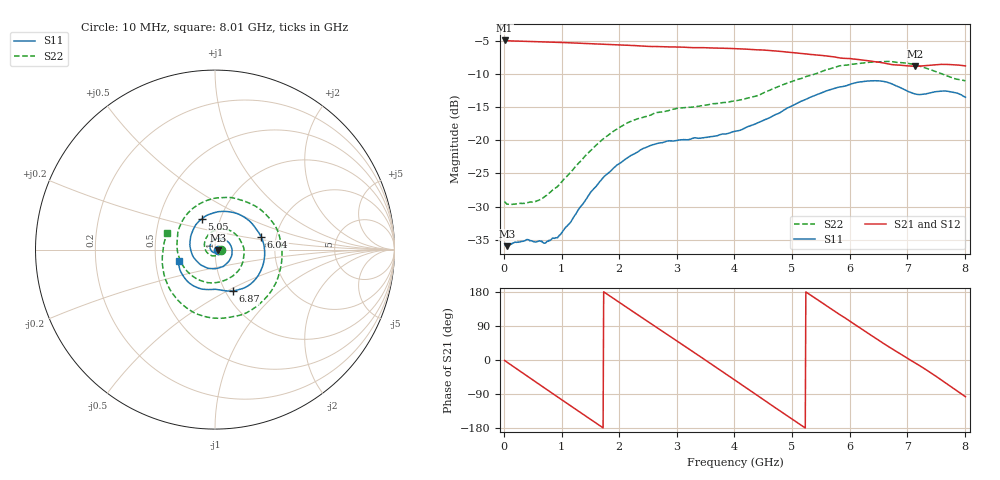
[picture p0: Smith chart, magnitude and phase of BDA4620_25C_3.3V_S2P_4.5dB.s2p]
!Agilent Technologies,E5071B,MY42404982,A.09.10
!Date: Wed May 06 08:56:56 2026
!Data & Calibration Information:
!Freq	S11:SOLT2(ON)	S21:SOLT2(ON)	S12:SOLT2(ON)	S22:SOLT2(ON)
# Hz S RI R 50
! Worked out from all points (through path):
!   801 points, 10 MHz to 8.01 GHz, reference 50 ohm
!   highest |S21| = -4.95 dB at 10 MHz (marker M1); lowest = -8.8 dB at 7.14 GHz (marker M2)
!   group delay of S21, straight-line fit = 283 ps
!   lowest |S11| = -36.0 dB at 60 MHz (marker M3), VSWR 1.03, Z = 51.6 - j0.143 ohm
!   |S11| at or under -10 dB: start of sweep to end of sweep
!   |S22| runs from -29.7 to -8.1 dB; largest |S21 - S12| = 0.0027
!   S11 on the Smith chart (normalised r, x): 10 MHz: 1.03, -0.00; 5.05 GHz: 0.82, +0.29; 6.04 GHz: 1.67, +0.26; 6.87 GHz: 1.08, -0.53; 8.01 GHz: 0.66, -0.08
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1e7  0.0166 -0.000983  0.5656 -0.0118  0.5661 -0.0123  0.0344 -0.00275
6e7  0.0158 -0.00139  0.5596 -0.0645  0.5608 -0.0654  0.0325 -0.0058
3.7e8  0.0143 -0.0101  0.4328 -0.3513  0.4332 -0.3522  0.0191 -0.0275
7.3e8  -8.32e-05 -0.017  0.1274 -0.5364  0.127 -0.5372  -0.0173 -0.0341
1.03e9  -0.0188 -0.00905  -0.1668 -0.5192  -0.1675 -0.5198  -0.0495 -0.0093
1.35e9  -0.0279 0.0165  -0.4186 -0.3392  -0.4189 -0.3394  -0.0573 0.0423
1.64e9  -0.0156 0.0447  -0.5251 -0.0844  -0.5256 -0.085  -0.0282 0.0909
1.93e9  0.0155 0.0614  -0.4913 0.1847  -0.4917 0.1851  0.0326 0.1147
2.32e9  0.0663 0.0476  -0.253 0.4497  -0.2537 0.4499  0.1226 0.078
2.68e9  0.0951 -0.000848  0.0618 0.5045  0.0626 0.505  0.162 -0.00966
3.38e9  0.0345 -0.0975  0.4891 0.102  0.4897 0.101  0.0451 -0.1747
3.69e9  -0.0225 -0.1055  0.4651 -0.1705  0.4647 -0.1718  -0.0666 -0.1771
4.01e9  -0.0835 -0.0815  0.2931 -0.3931  0.293 -0.3939  -0.1685 -0.1052
4.5e9  -0.1396 0.0215  -0.1169 -0.4644  -0.1177 -0.4651  -0.2069 0.0946
5.05e9  -0.0741 0.1707  -0.4315 -0.1481  -0.4322 -0.1476  -0.0186 0.2822
5.35e9  0.0276 0.2123  -0.4337 0.0889  -0.4336 0.0893  0.1408 0.2769
6.04e9  0.2571 0.0715  -0.0626 0.4067  -0.0621 0.4073  0.3734 -0.0199
6.68e9  0.1766 -0.2066  0.308 0.2144  0.3095 0.2142  0.1828 -0.3482
6.87e9  0.099 -0.2302  0.3518 0.1094  0.353 0.1085  0.0651 -0.3799
7.14e9  0.0164 -0.2227  0.3577 -0.0508  0.3582 -0.052  -0.1097 -0.3548
7.57e9  -0.109 -0.2071  0.2375 -0.2879  0.2377 -0.289  -0.2784 -0.1583
8.01e9  -0.2022 -0.0608  -0.0429 -0.3609  -0.0439 -0.3616  -0.2661 0.0904
